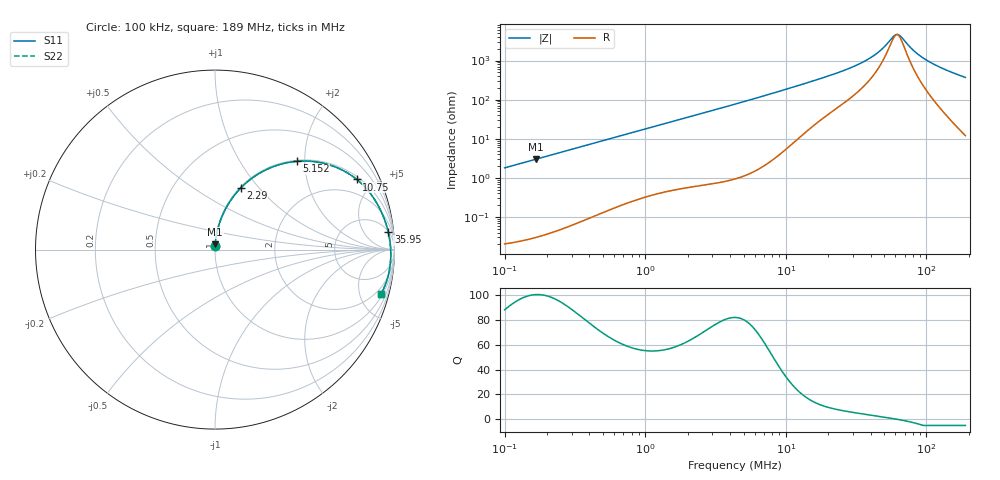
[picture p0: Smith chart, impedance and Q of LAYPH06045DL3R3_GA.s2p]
! LAYPH06045DL3R3_GA  S-PARAMETER MODEL  ( General Type )
! Model Generated by TAIYO YUDEN Corporation (http://www.ty-top.com)
! Version 2.0
! TAIYO YUDEN Control No. 180914NI43SB-FBB
! Copyright(c) 2018 TAIYO YUDEN CO.,LTD. All Rights Reserved.
! Product Description (link to TY-COMPAS)
! https://ds.yuden.co.jp/TYCOMPAS/or/detail?pn=LAYPH06045DL3R3NGA&u=M
! Products Name : Inductors
! Characteristics :
!  Inductance : 3.3 uH , SRF(min) : -Hz , DC Resistance(max) : 0.0195 Ohm
!  Rated Current : Saturation :3.5 A , Temp Rise : 2.5 A (25 degC)
!  Case Size : 6.3 x 6.0 / 0.248 x 0.236 [mm/inch] , Thickness : 4.5 / 0.177 [mm/inch]
!  (Conditions: Temperature = 25 degC , DC Bias Current/Voltage = 0A / 0V)
! External Node Assignments :
!  1  o---GGG---o  2
! GND o---------o GND
! Frequency Range : 0.1MHz  -  189.042664MHz  [ 402 STEP ]
# MHz S RI R 50
! Freq[MHz].  S11 Real  S11 Imag  S21 Real  S21 Imag  S12 Real  S12 Imag  S22 Real  S22 Imag
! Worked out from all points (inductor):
!   401 points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, 100 kHz to 189 MHz, reference 50 ohm
!   read as one part in series: L = 2.86 uH near 103.8 kHz
!   highest Q = 100 at 166.4 kHz (marker M1), where L = 2.86 uH
!   self-resonance near 61.51 MHz
!   S11 on the Smith chart (normalised r, x): 100 kHz: 1.00, +0.04; 2.29 MHz: 1.01, +0.80; 5.152 MHz: 1.02, +1.82; 10.75 MHz: 1.13, +3.97; 35.95 MHz: 5, +18; 189 MHz: 1.24, -7.38
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0.1  0.000527 0.018  0.9995 -0.018  0.9995 -0.018  0.000527 0.018
0.166406  0.00119 0.0298  0.9988 -0.0298  0.9988 -0.0298  0.00119 0.0298
0.353854  0.00477 0.0631  0.9952 -0.0631  0.9952 -0.0631  0.00477 0.0631
0.697773  0.0172 0.1219  0.9828 -0.1219  0.9828 -0.1219  0.0172 0.1219
1.252125  0.0501 0.2092  0.9499 -0.2092  0.9499 -0.2092  0.0501 0.2092
2.289667  0.1428 0.3424  0.8572 -0.3424  0.8572 -0.3424  0.1428 0.3424
4.347904  0.3713 0.4771  0.6287 -0.4771  0.6287 -0.4771  0.3713 0.4771
5.152316  0.4542 0.4916  0.5458 -0.4916  0.5458 -0.4916  0.4542 0.4916
7.235153  0.6251 0.4757  0.3749 -0.4757  0.3749 -0.4757  0.6251 0.4757
10.75145  0.7896 0.391  0.2104 -0.391  0.2104 -0.391  0.7896 0.391
15.38522  0.8816 0.2906  0.1184 -0.2906  0.1184 -0.2906  0.8816 0.2906
25.60186  0.9451 0.166  0.0549 -0.166  0.0549 -0.166  0.9451 0.166
35.95147  0.9657 0.0972  0.0343 -0.0972  0.0343 -0.0972  0.9657 0.0972
45.08307  0.9735 0.0553  0.0265 -0.0553  0.0265 -0.0553  0.9735 0.0553
54.44117  0.9774 0.0217  0.0226 -0.0217  0.0226 -0.0217  0.9774 0.0217
59.82524  0.9786 0.00495  0.0214 -0.00495  0.0214 -0.00495  0.9786 0.00495
63.30801  0.9791 -0.00514  0.0209 0.00514  0.0209 0.00514  0.9791 -0.00514
66.99353  0.9794 -0.0153  0.0206 0.0153  0.0206 0.0153  0.9794 -0.0153
80.89969  0.979 -0.0502  0.021 0.0502  0.021 0.0502  0.979 -0.0502
97.69241  0.9759 -0.0876  0.0241 0.0876  0.0241 0.0876  0.9759 -0.0876
132.1062  0.9625 -0.1548  0.0375 0.1548  0.0375 0.1548  0.9625 -0.1548
189.0427  0.9247 -0.2481  0.0753 0.2481  0.0753 0.2481  0.9247 -0.2481
